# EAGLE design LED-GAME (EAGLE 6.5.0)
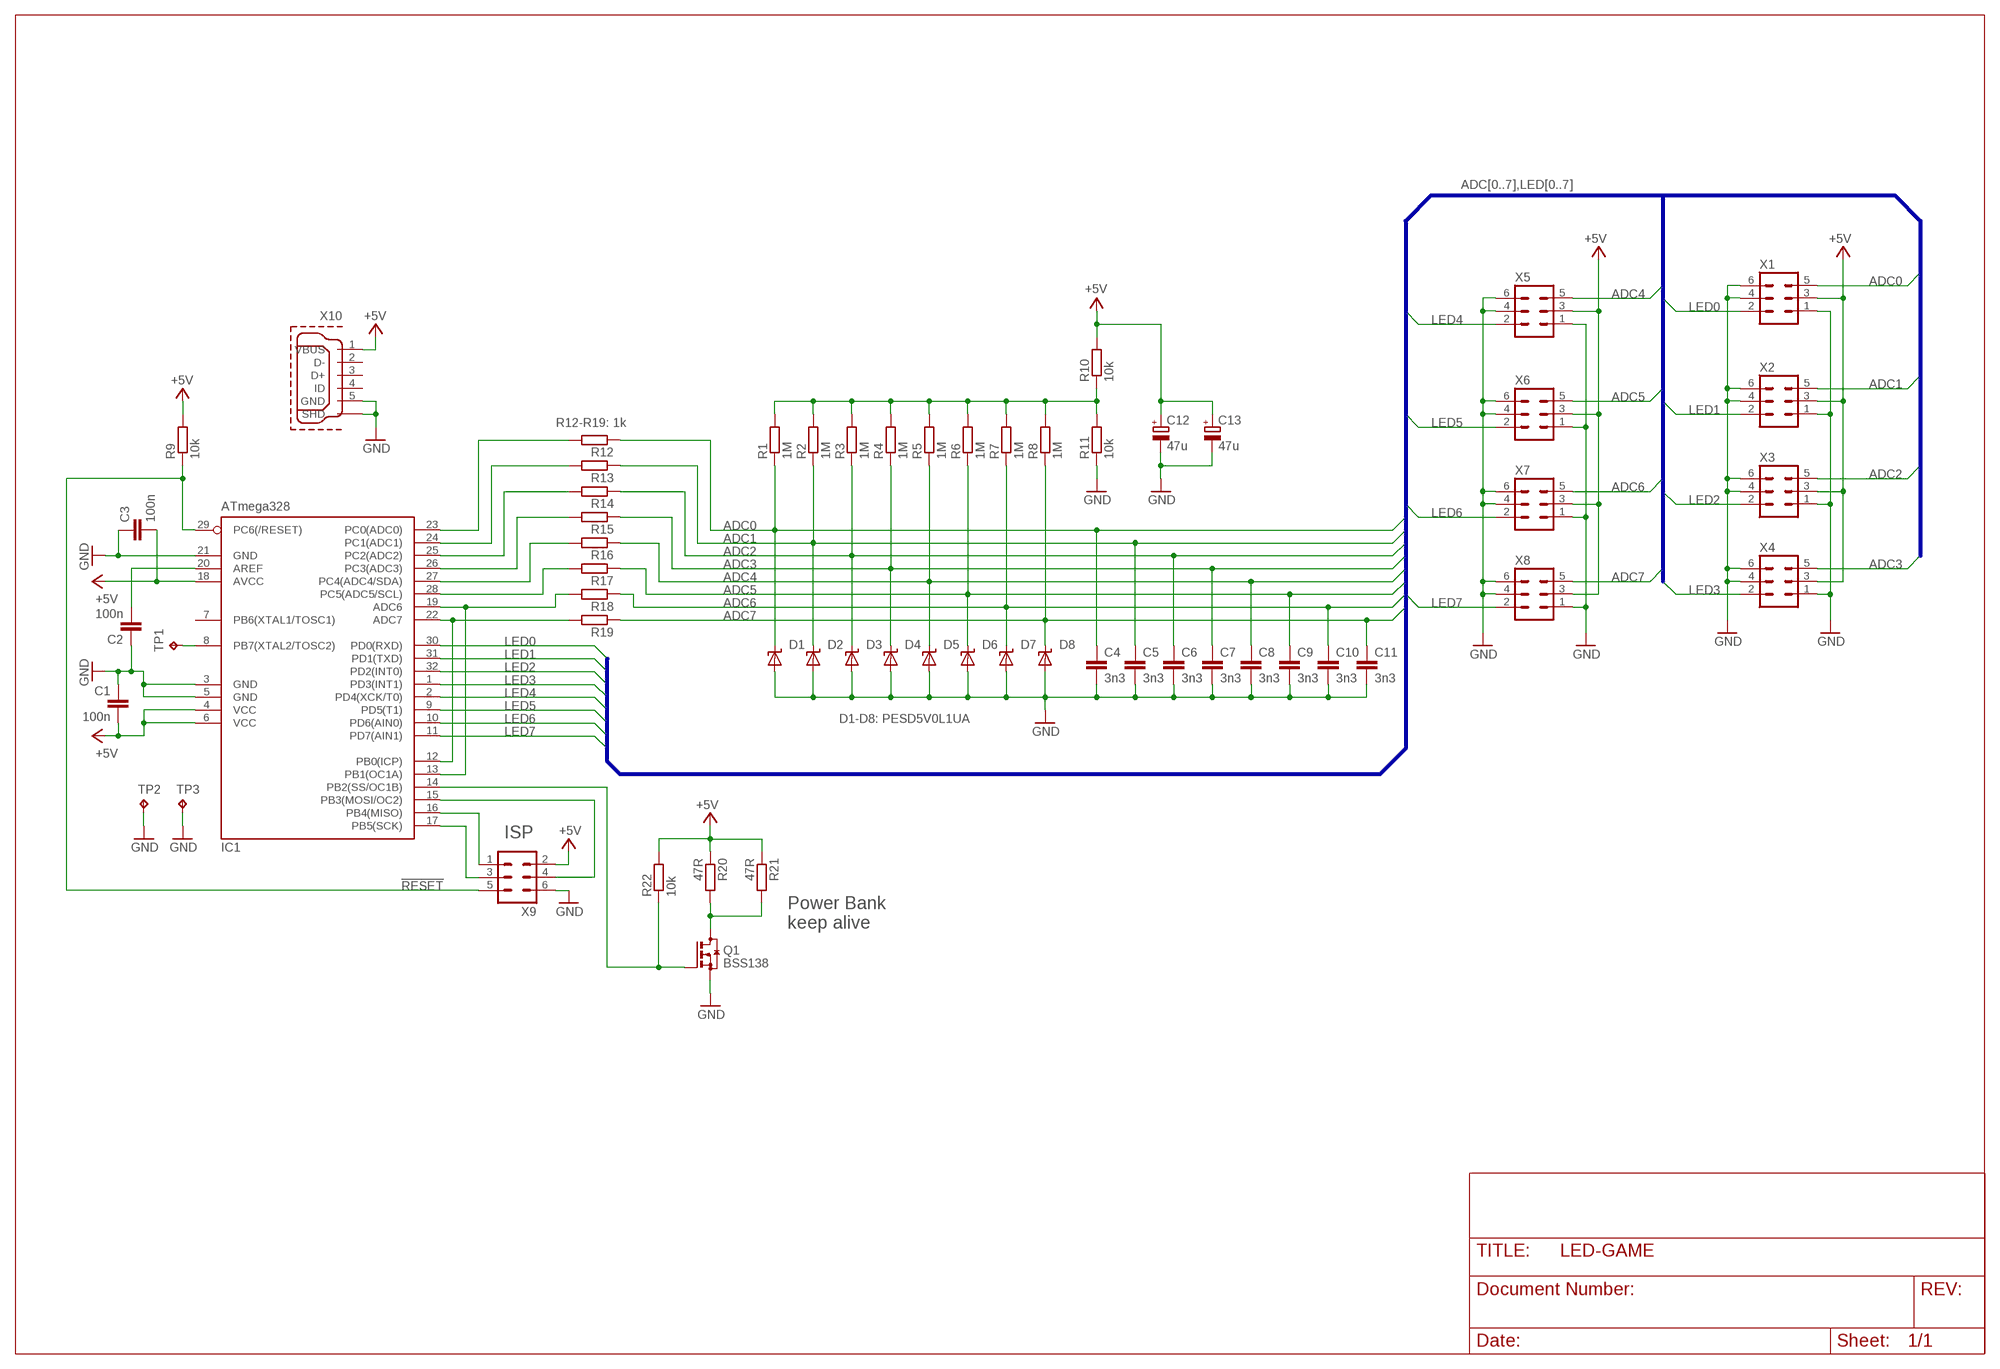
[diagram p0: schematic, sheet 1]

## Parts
C1  100n  C-EUC0603  [C0603]
C2  100n  C-EUC0603  [C0603]
C3  100n  C-EUC0603  [C0603]
C4  3n3  C-EUC0603K  [C0603K]
C5  3n3  C-EUC0603K  [C0603K]
C6  3n3  C-EUC0603K  [C0603K]
C7  3n3  C-EUC0603K  [C0603K]
C8  3n3  C-EUC0603K  [C0603K]
C9  3n3  C-EUC0603K  [C0603K]
C10  3n3  C-EUC0603K  [C0603K]
C11  3n3  C-EUC0603K  [C0603K]
C12  47u  CPOL-EUB/3528-21R  [B/3528-21R]
C13  47u  CPOL-EUB/3528-21R  [B/3528-21R]
D1  PESD5V  SUPPRESSOR_UNI  [SOD323-W]
D2  PESD5V  SUPPRESSOR_UNI  [SOD323-W]
D3  PESD5V  SUPPRESSOR_UNI  [SOD323-W]
D4  PESD5V  SUPPRESSOR_UNI  [SOD323-W]
D5  PESD5V  SUPPRESSOR_UNI  [SOD323-W]
D6  PESD5V  SUPPRESSOR_UNI  [SOD323-W]
D7  PESD5V  SUPPRESSOR_UNI  [SOD323-W]
D8  PESD5V  SUPPRESSOR_UNI  [SOD323-W]
IC1  ATmega328  MEGA8-AI  [TQFP32-08]
Q1  BSS138  BSS123  [SOT23]
R1  1M  R-EU_R0603  [R0603]
R2  1M  R-EU_R0603  [R0603]
R3  1M  R-EU_R0603  [R0603]
R4  1M  R-EU_R0603  [R0603]
R5  1M  R-EU_R0603  [R0603]
R6  1M  R-EU_R0603  [R0603]
R7  1M  R-EU_R0603  [R0603]
R8  1M  R-EU_R0603  [R0603]
R9  10k  R-EU_R0603  [R0603]
R10  10k  R-EU_R0603  [R0603]
R11  10k  R-EU_R0603  [R0603]
R12  1k  R-EU_R0603  [R0603]
R13  1k  R-EU_R0603  [R0603]
R14  1k  R-EU_R0603  [R0603]
R15  1k  R-EU_R0603  [R0603]
R16  1k  R-EU_R0603  [R0603]
R17  1k  R-EU_R0603  [R0603]
R18  1k  R-EU_R0603  [R0603]
R19  1k  R-EU_R0603  [R0603]
R20  47R  R-EU_R1206  [R1206]
R21  47R  R-EU_R1206  [R1206]
R22  10k  R-EU_R0603  [R0603]
TP1  TPP1-08  [P1-08]
TP2  TPP1-08  [P1-08]
TP3  TPP1-08  [P1-08]
X1  ML6  [ML6]
X2  ML6  [ML6]
X3  ML6  [ML6]
X4  ML6  [ML6]
X5  ML6  [ML6]
X6  ML6  [ML6]
X7  ML6  [ML6]
X8  ML6  [ML6]
X9  ML6  [ML6]
X10  MOLEX-1051330001MOD  [MOLEX_1051330001-MOD]

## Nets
!RESET: IC1.29(PC6(/RESET)) R9.1 X9.5
+5V: C1.2 C3.2 C12.+ C13.+ IC1.4(VCC) IC1.6(VCC) IC1.18(AVCC) R9.2 R10.2 R20.1 R21.1 R22.2 X1.3 X2.3 X3.3 X4.3 X5.3 X6.3 X7.3 X8.3 X9.2 X10.1(VBUS)
ADC0: C4.1 D1.C R1.1 R12.1 X1.5
ADC1: C5.1 D2.C R2.1 R13.1 X2.5
ADC2: C6.1 D3.C R3.1 R14.1 X3.5
ADC3: C7.1 D4.C R4.1 R15.1 X4.5
ADC4: C8.1 D5.C R5.1 R16.1 X5.5
ADC5: C9.1 D6.C R6.1 R17.1 X6.5
ADC6: C10.1 D7.C R7.1 R18.1 X7.5
ADC7: C11.1 D8.C R8.1 R19.1 X8.5
GND: C1.1 C2.1 C3.1 C4.2 C5.2 C6.2 C7.2 C8.2 C9.2 C10.2 C11.2 C12.- C13.- D1.A D2.A D3.A D4.A D5.A D6.A D7.A D8.A IC1.3(GND) IC1.5(GND) IC1.21(GND) Q1.2(S) R11.1 TP2.TP TP3.TP X1.1 X1.4 X1.6 X2.1 X2.4 X2.6 X3.1 X3.4 X3.6 X4.1 X4.4 X4.6 X5.1 X5.4 X5.6 X6.1 X6.4 X6.6 X7.1 X7.4 X7.6 X8.1 X8.4 X8.6 X9.6 X10.5(GND) X10.P$1(SHD) X10.P$2(SHD) X10.P$3(SHD) X10.P$5(SHD) X10.P$6(SHD) X10.P$9(SHD)
LED0: IC1.30(PD0(RXD)) X1.2
LED1: IC1.31(PD1(TXD)) X2.2
LED2: IC1.32(PD2(INT0)) X3.2
LED3: IC1.1(PD3(INT1)) X4.2
LED4: IC1.2(PD4(XCK/T0)) X5.2
LED5: IC1.9(PD5(T1)) X6.2
LED6: IC1.10(PD6(AIN0)) X7.2
LED7: IC1.11(PD7(AIN1)) X8.2
N$1: C2.2 IC1.20(AREF)
N$2: IC1.8(PB7(XTAL2/TOSC2)) TP1.TP
N$3: IC1.23(PC0(ADC0)) R12.2
N$4: R1.2 R2.2 R3.2 R4.2 R5.2 R6.2 R7.2 R8.2 R10.1 R11.2
N$5: IC1.24(PC1(ADC1)) R13.2
N$6: IC1.16(PB4(MISO)) X9.1
N$7: IC1.17(PB5(SCK)) X9.3
N$8: IC1.26(PC3(ADC3)) R15.2
N$9: IC1.25(PC2(ADC2)) R14.2
N$10: IC1.27(PC4(ADC4/SDA)) R16.2
N$11: IC1.15(PB3(MOSI/OC2)) X9.4
N$12: IC1.28(PC5(ADC5/SCL)) R17.2
N$13: IC1.14(PB2(SS/OC1B)) Q1.1(G) R22.1
N$14: Q1.3(D) R20.2 R21.2
N$15: IC1.12(PB0(ICP)) IC1.22(ADC7) R19.2
N$16: IC1.13(PB1(OC1A)) IC1.19(ADC6) R18.2
Unconnected: IC1.7(PB6(XTAL1/TOSC1)) X10.2(D-) X10.3(D+) X10.4(ID)

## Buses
ADC[0..7],LED[0..7]

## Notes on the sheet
- R12-R19: 1k
- D1-D8: PESD5V0L1UA
- ISP
- Power Bank
  keep alive

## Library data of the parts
C1-C11 = rcl:C-EU: CAPACITOR, European symbol
C12 C13 = rcl:CPOL-EU: POLARIZED CAPACITOR, European symbol
D1-D8 = Brunner:SUPPRESSOR_UNI
IC1 = atmel:MEGA8: MICROCONTROLLER 8 Kbytes FLASH, 1 kbytes SRAM, 512 bytes EEPROM, USART, 6-channel 10 bit ADC, 2-channel 8 bit ADC Pin compatible with Atmega48, ATMega88, ATMega168 Source: avr.lbr; MPN: ATMEGA8-16AU; OC_FARNELL: 9171371; OC_NEWARK: 73M8863
Q1 = transistor-small-signal:BSS123: N-CHANNEL MOS FET
R1-R22 = rcl:R-EU_: RESISTOR, European symbol
TP1-TP3 = testpad:TP: Test pad
X1-X9 = con-harting-ml:ML6: HARTING; OC_FARNELL: unknown; OC_NEWARK: unknown
X10 = Langloch_cherry:MOLEX-1051330001: USB - Mikro-B Buchsenleiste Steckverbinder 5 Positionen Oberflächenmontage, vertikal

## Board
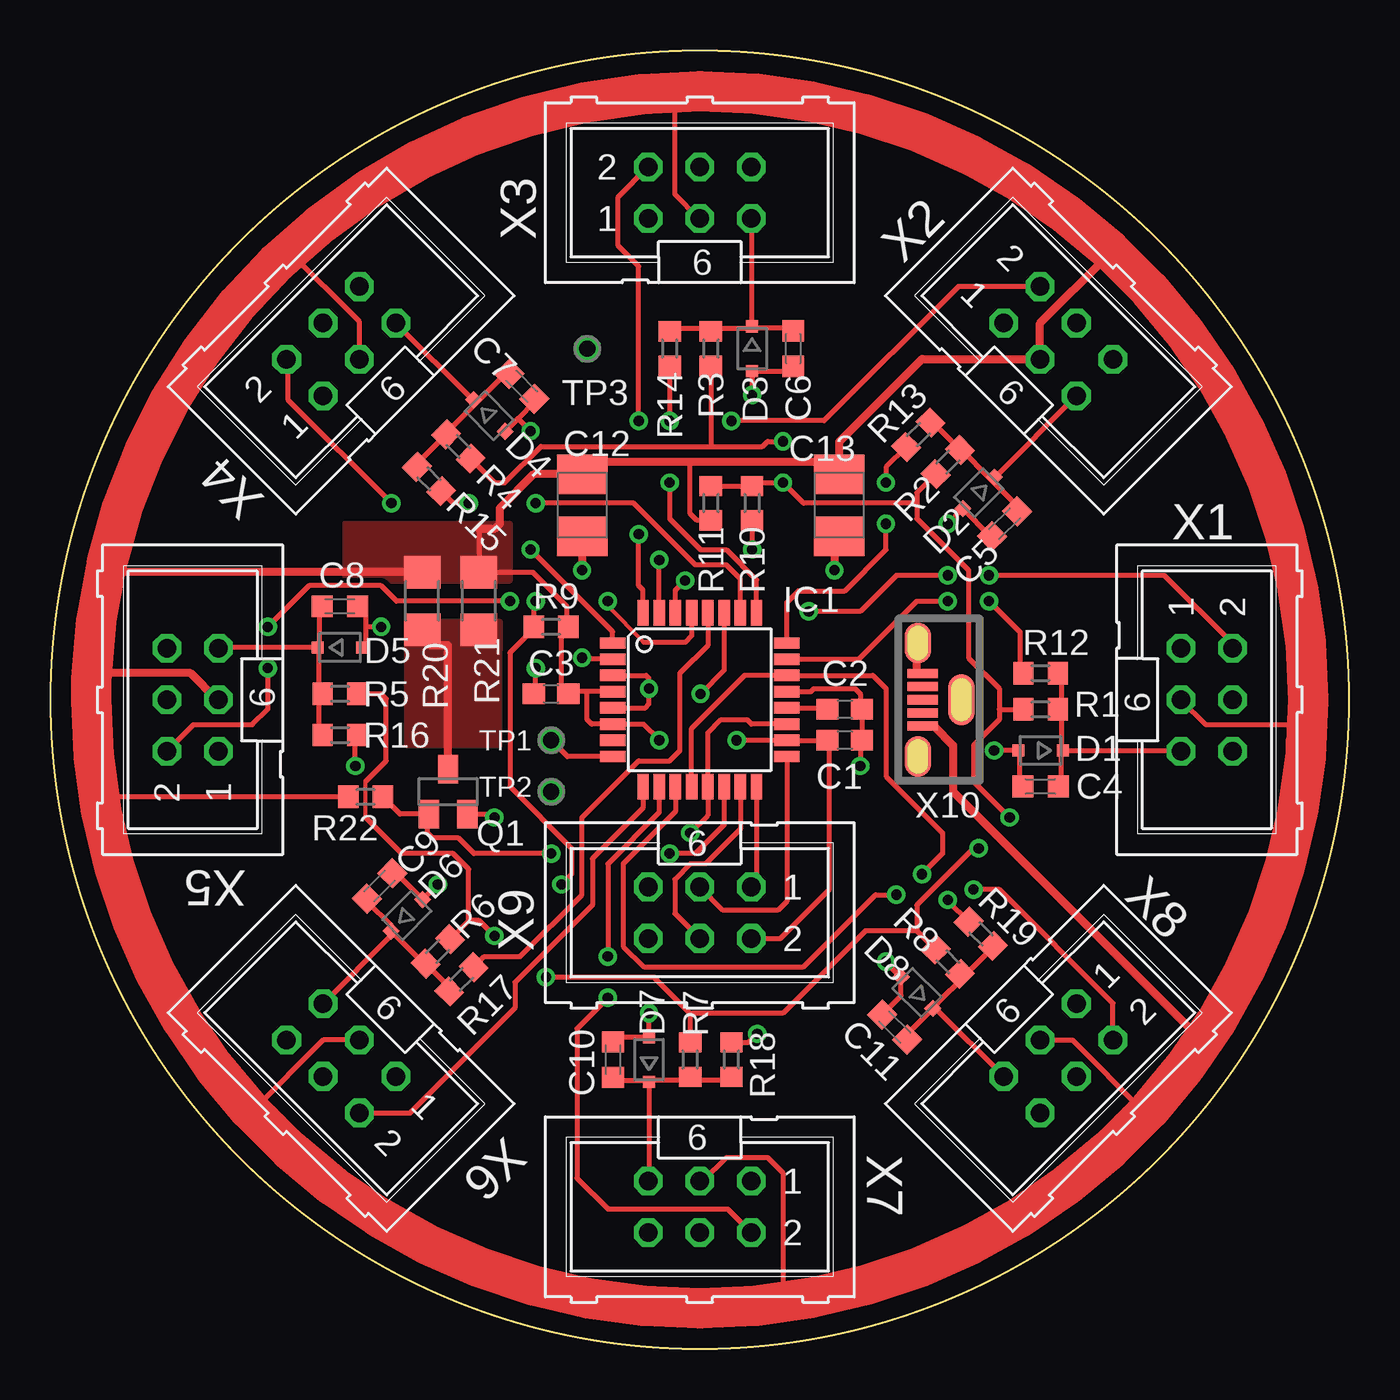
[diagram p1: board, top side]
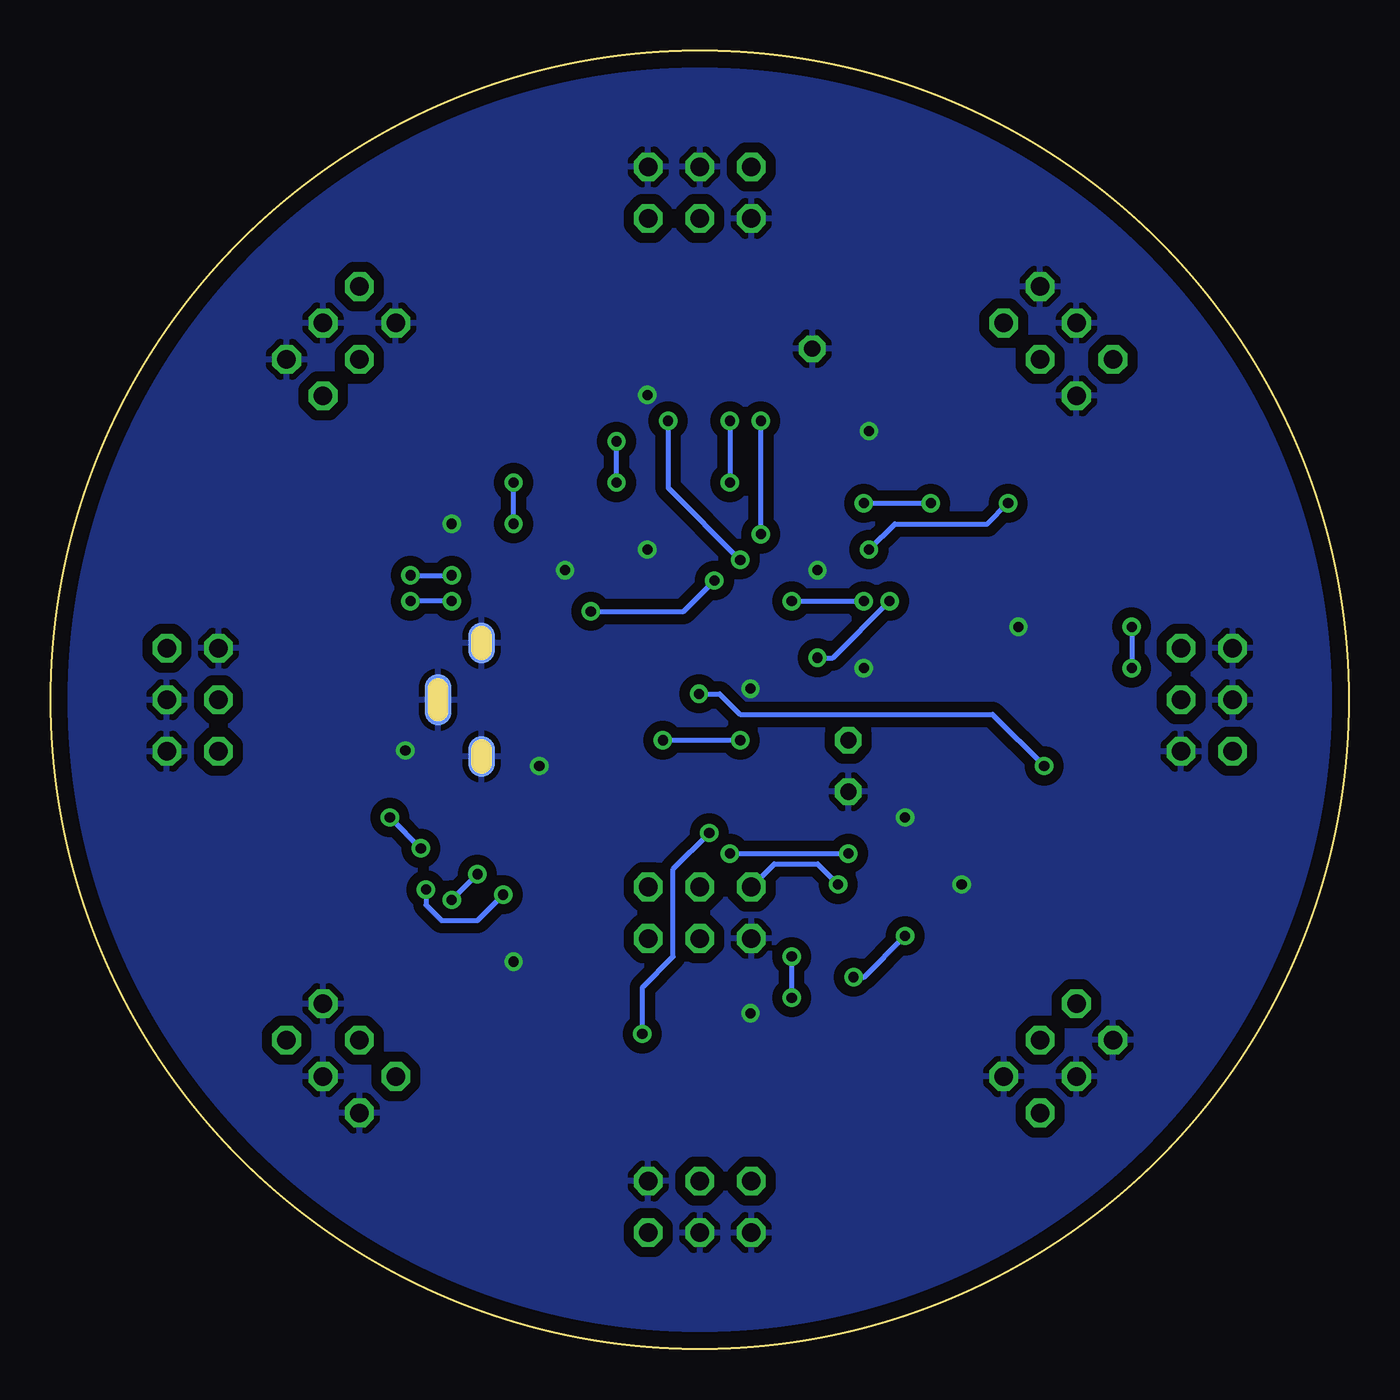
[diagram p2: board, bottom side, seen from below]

Size 64 x 64 mm. Coordinates in mm from the lower left corner, seen from the top.
Outline: circle at 32,32 radius 32
Copper layers (1*16): Top 0.035mm / dielectric 1.5mm / Bottom 0.035mm
Design rules "default *": minimum track width 0.25mm, minimum drill 0.5mm, track to track 0.25mm, track to pad 0.25mm, pad to pad 0.22mm, via to via 0.3mm, smd to smd 8mil, copper to edge 0.8mm, drill to drill 8mil, minimum pad ring 10mil, minimum via ring 8mil, stop-mask expansion 4mil, vias tented up to drill 0mil, thermal gap 0.3mm
bRestrict: 4 lines

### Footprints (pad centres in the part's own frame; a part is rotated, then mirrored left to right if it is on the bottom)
C0603 = smd 1.1 x 1: 1 -0.85,0; 2 0.85,0
C0603K = smd 1.05 x 1.08: 1 -0.875,0; 2 0.875,0
B/3528-21R = smd 1.95 x 2.5: + 1.525,0; - -1.525,0
SOD323-W = smd 0.6 x 0.6: A 1.1,0; C -1.1,0
TQFP32-08 = smd 1.27 x 0.559: 1 -4.293,2.8; 2 -4.293,2; 3 -4.293,1.2; 4 -4.293,0.4; 5 -4.293,-0.4; 6 -4.293,-1.2; 7 -4.293,-2; 8 -4.293,-2.8; 17 4.293,-2.8; 18 4.293,-2; 19 4.293,-1.2; 20 4.293,-0.4; 21 4.293,0.4; 22 4.293,1.2; 23 4.293,2; 24 4.293,2.8 | smd 0.559 x 1.27: 9 -2.8,-4.293; 10 -2,-4.293; 11 -1.2,-4.293; 12 -0.4,-4.293; 13 0.4,-4.293; 14 1.2,-4.293; 15 2,-4.293; 16 2.8,-4.293; 25 2.8,4.293; 26 2,4.293; 27 1.2,4.293; 28 0.4,4.293; 29 -0.4,4.293; 30 -1.2,4.293; 31 -2,4.293; 32 -2.8,4.293
SOT23 = smd 1 x 1.4: 1 -0.95,-1.1; 2 0.95,-1.1; 3 0,1.1
R0603 = smd 1 x 1.1: 1 -0.85,0; 2 0.85,0
R1206 = smd 1.6 x 1.803: 1 -1.422,0; 2 1.422,0
P1-08 = drill 0.8 octagon: TP 0,0
ML6 = drill 0.914 octagon: 1 -2.54,-1.27; 2 -2.54,1.27; 3 0,-1.27; 4 0,1.27; 5 2.54,-1.27; 6 2.54,1.27
MOLEX_1051330001-MOD = smd 1.5 x 0.45: 1 0,1.3; 2 0,0.65; 3 0,0; 4 0,-0.65; 5 0,-1.3 | smd 1.3 x 2 bottom: P$1 0.24,-2.8; P$9 0.24,2.8 | smd 1.3 x 2: P$2 0.24,-2.8; P$3 0.24,2.8 | smd 1.3 x 2.5: P$5 -1.9,0 | smd 1.3 x 2.5 bottom: P$6 -1.9,0

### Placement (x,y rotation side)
C1  39.15,30.01 180 top
C2  39.15,31.53 180 top
C3  24.67,32.29 0 top
C4  48.8,27.72 180 top
C5  47.02,40.67 225 top
C6  36.61,49.31 270 top
C7  23.22,47.46 315 top
C8  14.26,36.61 0 top
C9  16.22,22.82 45 top
C10  27.72,14.26 90 top
C11  41.62,15.86 135 top
C12  26.22,41.59 90 top
C13  38.88,41.59 90 top
D1  48.8,29.5 180 top
D2  45.75,42.2 225 top
D3  34.58,49.31 270 top
D4  21.62,46.01 315 top
D5  14.26,34.58 0 top
D6  17.56,21.37 45 top
D7  29.5,14.26 90 top
D8  42.71,17.56 135 top
IC1  32,32 0 top
Q1  19.59,27.47 0 top
R1  48.8,31.53 180 top
R2  44.23,43.72 225 top
R3  32.55,49.31 270 top
R4  20.1,44.48 315 top
R5  14.26,32.29 0 top
R6  19.08,19.59 45 top
R7  31.53,14.26 90 top
R8  44.23,19.08 135 top
R9  24.67,35.59 0 top
R10  32.55,41.69 270 top
R11  34.58,41.69 90 top
R12  48.8,33.31 180 top
R13  42.78,45.07 225 top
R14  30.51,49.31 270 top
R15  18.65,42.89 315 top
R16  14.26,30.26 0 top
R17  20.25,18.22 45 top
R18  33.56,14.26 90 top
R19  45.86,20.46 135 top
R20  18.32,36.86 270 top
R21  21.12,36.86 270 top
R22  15.53,27.21 180 top
TP1  24.67,30.01 0 top
TP2  24.67,27.47 0 top
TP3  26.45,49.31 0 top
X1  57,32 270 top
X2  49.68,49.68 315 top
X3  32,57 0 top
X4  14.32,49.68 45 top
X5  7,32 90 top
X6  14.32,14.32 135 top
X7  32,7 180 top
X8  49.68,14.32 225 top
X9  32,21.5 180 top
X10  43,32 180 top

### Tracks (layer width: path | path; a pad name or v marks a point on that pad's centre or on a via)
!RESET  (via drill 0.5)
  Top 0.2: 29.24,34.83 27.47,36.61
  Top 0.254: IC1.29 31.6,35.16 31.28,34.83 29.24,34.83 | 27.47,36.61 v27.47,36.86 | v23.91,36.86 23.82,36.78 R9.1 23.82,35.51 22.64,34.32 22.64,27.72 25.69,24.67 25.69,23.4 v25.18,22.89
  Bottom 0.254: v27.47,36.86 v23.91,36.86 | v25.18,22.89 26.2,23.91 28.32,23.91 X9.5
+5V  (via drill 0.5)
  Top 0.254: IC1.4 26.45,32.4 | 26.45,32.4 25.63,32.4 | 25.63,32.4 C3.2 | 26.45,32.4 26.45,31.02 26.67,30.8 IC1.6 29.21,30.8 v30.01,30.01 | C12.+ 26.31,43.21 26.45,43.21 26.96,43.72 | 21.12,40.42 R21.1 23.76,38.29 25.43,36.61 25.43,35.68 R9.2 25.18,35.25 25.18,32.55 25.33,32.4 25.63,32.4 | C13.+ 38.88,43.23 38.39,43.72 | v33.82,30.01 v33.82,30 IC1.18 C1.2 38.39,29.92 38.39,22.64 35.98,20.23 X9.2 | X7.3 32.15,8.27 33.31,9.43 35.34,9.43 36.1,8.67 36.1,2.83 36.36,2.57 32.57,2.57 32,2 | X6.3 13.44,15.22 9.94,11.72 9.94,12.48 6.64,15.78 6.64,16.8 4.35,19.08 4.35,22.13 3.08,23.4 3.08,25.69 2.07,26.7 2.07,27.21 | 2.07,27.21 2.07,31.93 2,32 | X4.3 15.22,50.63 11.72,54.14 12.73,54.14 17.31,58.71 19.08,58.71 20.61,60.23 23.4,60.23 24.67,61.5 28.99,61.5 29.24,61.76 30.77,61.76 | 30.77,61.76 31.76,61.76 32,62 32.24,61.76 37.88,61.76 38.9,60.74 41.44,60.74 42.96,59.22 44.99,59.22 46.52,57.69 48.04,57.69 51.85,53.88 52.1,53.88 | X3.3 31.97,55.73 30.77,56.93 30.77,61.76 | 62.01,32.8 62.01,32.01 62,32 62,31.01 61.76,30.77 | R10.2 31.87,40.84 31.53,41.18 31.53,43.72 | R22.2 2.07,27.21 | X1.3 56.96,30.77 61.76,30.77 | 61.76,30.77 60.99,30.01 60.99,24.93 59.98,23.91 59.98,23.4 | 59.98,22.39 59.47,21.88 59.47,19.59 58.71,18.83 58.71,18.07 57.44,16.8 57.44,16.04 56.68,15.27 55.91,14.51 55.91,13.5 54.14,11.72 53.88,11.72 50.38,15.22 X8.3
  Top 0.406: C12.+ 23.81,43.12 22.13,41.44 22.13,40.67 21.88,40.42 21.12,40.42 | 38.39,43.72 31.53,43.72 26.96,43.72 | R20.1 2.68,38.29 2.57,38.39 2.57,33.57 | 2.57,33.57 2,33 | X5.3 8.2,32 6.89,33.31 2.84,33.31 2.57,33.57 | X2.3 48.78,50.56 52.1,53.88 | 59.98,22.39 59.98,23.4 | 56.68,15.27 44.48,27.47 44.48,29.75 43.54,30.7 X10.1 | C13.+ 38.88,44.72 42.96,48.8 48.8,48.8
  Top 2: 2,32 2,33 arc-88 32,62 arc-90 62,32 arc-90 32,2 arc-90 2,32
  Bottom 0.254: v33.82,30.01 v30.01,30.01
  pour Top (no thermals): 22.64,40.67 14.51,40.67 14.51,37.88 22.64,37.88
ADC0
  Top 0.254: R12.1 49.82,33.31 49.82,31.7 R1.1 49.82,31.53 49.82,29.58 D1.C | D1.C 55.69,29.5 X1.5 | C4.1 49.68,27.83 49.82,27.97 49.82,29.41 D1.C
ADC1
  Top 0.254: R13.1 43.47,45.75 43.47,45.69 R2.1 44.9,44.32 46.26,42.96 | 46.26,42.96 46.52,42.96 D2.C 46.57,42.98 X2.5 | C5.1 47.64,41.58 46.26,42.96
ADC2
  Top 0.254: D3.C 34.58,55.69 X3.5 | R14.1 30.51,50.33 32.38,50.33 R3.1 32.55,50.33 34.49,50.33 D3.C | C6.1 36.61,50.33 34.66,50.33 D3.C
ADC3
  Top 0.254: R15.1 18.05,43.7 18.07,43.72 18.14,43.72 R4.1 19.5,45.15 20.86,46.52 | 20.86,46.52 20.86,46.77 D4.C 20.81,46.79 X4.5 | C7.1 22.42,48.08 20.86,46.52
ADC4
  Top 0.254: 13.5,36.61 C8.1 13.24,36.61 13.24,34.66 D5.C | R16.1 13.41,30.35 13.24,30.51 13.24,32.13 R5.1 13.41,32.38 13.24,32.55 13.24,34.49 D5.C | D5.C 8.31,34.58 X5.5
ADC5
  Top 0.254: R17.1 19.85,17.81 19.66,17.81 R6.1 18.38,18.99 D6.C | C9.1 15.6,22.06 16.8,20.86 16.8,20.61 D6.C | D6.C 16.78,20.37 X6.5
ADC6
  Top 0.254: R18.1 33.56,13.24 31.7,13.24 R7.1 31.44,13.41 31.28,13.24 29.58,13.24 D7.C | C10.1 27.83,13.38 27.97,13.24 29.41,13.24 D7.C | D7.C 29.5,8.31 X7.5
ADC7
  Top 0.254: R19.1 46.46,19.65 46.52,19.59 46.26,19.59 45.25,18.58 44.92,18.58 R8.1 | R8.1 | R8.1 44.99,18.32 43.72,17.05 43.72,17.02 D8.C | C11.1 42.23,15.49 42.2,15.53 42.23,15.53 D8.C | D8.C 43.63,16.78 X8.5
GND  (via drill 0.5)
  Top 0.254: C4.2 47.79,27.72 47.79,29.41 D1.A v46.52,29.5 | v29.5,16.54 D7.A 27.72,15.36 C10.2 | C9.2 17.05,23.44 D6.A v19.08,22.89 | C8.2 15.53,36.61 15.53,35.59 | 15.53,35.59 15.53,34.76 15.36,34.76 D5.A | IC1.3 29.35,33.2 29.5,33.05 v29.5,32.55 29.5,31.78 29.31,31.6 IC1.5 | C3.1 23.82,32.46 23.91,32.55 v23.91,33.56 | C12.- 26.22,39.93 26.2,39.91 | C13.- 38.8,40.07 38.64,39.91 | R11.1 v34.58,39.4 | Q1.2 21.71,26.37 v21.88,26.2 | IC1.21 37.48,32.4 37.63,32.55 39.66,32.55 39.91,32.29 39.91,31.62 C2.1 C1.1 39.91,30.01 v39.91,28.74 | v34.58,47.02 D3.A 36.38,48.21 C6.2 | C5.2 46.34,40.05 D2.A v44.23,40.67 | v16.29,35.59 15.53,35.59 | C11.2 41.93,17.41 D8.A 41.91,18.32 41.18,19.05 v41.18,19.08 | C7.2 23.84,46.67 23.04,45.87 | 23.04,45.87 D4.A | X10.5 42.71,33.3 42.71,33.31 | v23.66,45.25 | v23.66,45.25 23.04,45.87
  Top 0.406: 26.2,39.91 v26.2,38.39 | 38.64,39.91 v38.64,38.39 | 42.71,33.31 42.71,34.75 X10.P$1
  pour Bottom (isolate 0.5): -5.3,69.63 69.63,69.63 69.63,-5.3 -5.3,-5.3
LED0  (via drill 0.5)
  Top 0.254: X1.2 58.27,34.76 54.9,38.13 v46.26,38.13 | v44.23,38.13 41.69,38.13 39.91,36.36 v37.37,36.36 | IC1.30 30.8,37.4 v31.28,37.88
  Bottom 0.254: v46.26,38.13 v44.23,38.13 | v37.37,36.36 32.8,36.36 v31.28,37.88
LED1  (via drill 0.5)
  Top 0.254: X2.2 44.75,52.37 38.13,45.75 v33.56,45.75 | IC1.31 v30,38.89 v30.01,38.9
  Bottom 0.254: v33.56,45.75 33.56,42.45 v30.01,38.9
LED2  (via drill 0.5)
  Top 0.254: IC1.32 29.2,37.42 28.99,37.63 v28.99,40.17 | v28.99,45.75 28.99,53.37 27.97,54.39 27.97,56.78 X3.2
  Bottom 0.254: v28.99,40.17 v28.99,45.75
LED3  (via drill 0.5)
  Top 0.254: IC1.1 27.71,35.35 v23.66,39.4 | v16.8,41.69 11.72,46.77 11.72,48.69 X4.2
  Bottom 0.254: v23.66,39.4 22.39,40.67 17.81,40.67 v16.8,41.69
LED4  (via drill 0.5)
  Top 0.254: IC1.2 26.27,34 v26.2,34.07 | X5.2 7.04,30.77 9.94,30.77 10.7,31.53 v10.7,33.56 | v22.64,36.86 17.05,36.86 16.29,37.63 12.73,37.63 v10.7,35.59
  Bottom 0.254: v26.2,34.07 25.43,34.07 v22.64,36.86 | v10.7,35.59 v10.7,33.56
LED5
  Top 0.254: IC1.9 29.2,26.66 26.7,24.16 26.7,21.88 22.89,18.07 22.89,16.8 17.72,11.63 X6.2
LED6  (via drill 0.5)
  Top 0.254: IC1.10 30,26.44 27.47,23.91 v27.47,19.34 | v27.47,17.31 25.94,15.78 25.94,8.42 27.47,6.89 33.38,6.89 X7.2
  Bottom 0.254: v27.47,19.34 v27.47,17.31
LED7  (via drill 0.5)
  Top 0.254: X8.2 52.37,17.04 46.77,22.64 v45.5,22.64 | IC1.11 30.8,26.48 28.23,23.91 28.23,19.85 29.24,18.83 37.12,18.83 40.67,22.39 v41.69,22.39
  Bottom 0.254: v45.5,22.64 45.5,21.88 44.74,21.12 42.96,21.12 v41.69,22.39
N$1
  Top 0.254: IC1.20 38.23,31.6 C2.2
N$2
  Top 0.254: IC1.8 25.48,29.2 TP1.TP
N$3  (via drill 0.5)
  Top 0.254: IC1.23 39.84,34 42.71,36.86 v44.23,36.86 | v46.26,36.86 47.79,35.34 47.79,33.47 R12.2
  Bottom 0.254: v44.23,36.86 v46.26,36.86
N$4  (via drill 0.5)
  Top 0.2: 15.53,26.2 15.53,27.97
  Top 0.254: R10.1 R11.2 34.67,42.54 34.83,42.71 v36.1,42.71 37.12,41.69 42.71,41.69 | R3.2 32.55,44.48 | 32.55,44.48 35.09,44.48 35.34,44.74 v36.1,44.74 | R2.2 42.71,42.2 42.71,41.69 | 42.71,41.69 42.71,40.93 45.25,38.39 45.25,34.07 46.77,32.55 46.77,31.53 | 42.71,20.61 42.71,21.88 45.5,24.67 v45.75,24.67 | 42.71,20.61 R8.2 | 42.71,20.61 40.17,20.61 36.1,16.54 31.53,16.54 | 31.53,16.54 R7.2 | 31.53,16.54 29.75,18.32 v24.42,18.32 | v21.88,20.35 21.12,21.12 20.61,21.12 | 20.61,21.12 R6.2 | 20.61,21.12 20.61,23.66 19.85,24.42 17.31,24.42 15.53,26.2 | 15.53,27.97 16.54,28.99 16.54,32.04 16.29,32.29 R5.2 | R4.2 | R4.2 21.88,42.71 22.39,42.71 24.16,44.48 32.55,44.48 | 46.77,31.53 R1.2 | 46.77,31.53 46.77,31.02 45.5,29.75 45.5,27.97 v47.28,26.2
  Bottom 0.254: v36.1,42.71 v36.1,44.74 | v24.42,18.32 23.91,18.32 v21.88,20.35 | v47.28,26.2 v45.75,24.67
N$5  (via drill 0.5)
  Top 0.254: IC1.24 36.29,36.8 36.86,37.37 39.15,37.37 41.18,39.4 v41.18,40.67 | R13.2 41.18,43.47 v41.18,42.71
  Bottom 0.254: v41.18,40.67 v41.18,42.71
N$6
  Top 0.254: IC1.16 34.8,23.03 X9.1
N$7
  Top 0.254: IC1.17 36.29,22.07 35.85,21.62 33.15,21.62 X9.3
N$8  (via drill 0.5)
  Top 0.254: IC1.26 34,37.95 33.31,38.64 31.78,38.64 28.74,41.69 v23.91,41.69 | v20.61,41.69 19.85,41.69 R15.2
  Bottom 0.254: v23.91,41.69 v20.61,41.69
N$9  (via drill 0.5)
  Top 0.254: R14.2 v30.51,45.75 | v30.51,42.71 30.51,40.93 32.04,39.4 33.31,39.4 34.8,37.91 IC1.25
  Bottom 0.254: v30.51,45.75 v30.51,42.71
N$10  (via drill 0.5)
  Top 0.254: IC1.27 33.2,33.45 v32.04,32.29 | v15.02,28.74 15.02,30.17 R16.2
  Bottom 0.254: v32.04,32.29 31.02,32.29 30.01,31.28 17.56,31.28 v15.02,28.74
N$11
  Top 0.254: IC1.15 34,25.62 32.29,23.91 31.53,23.91 30.77,23.15 30.77,21.46 X9.4
N$12
  Top 0.254: IC1.28 32.4,34.69 31.02,33.31 31.02,29.5 30.51,28.99 28.99,28.99 26.2,26.2 26.2,22.39 23.15,19.34 21.37,19.34 R17.2
N$13  (via drill 0.5)
  Top 0.254: R22.1 17.22,26.37 Q1.1 18.58,26.3 18.58,25.43 18.83,25.18 20.1,25.18 20.86,24.42 v24.67,24.42 | IC1.14 33.2,25.83 31.78,24.42 v30.51,24.42
  Bottom 0.254: v30.51,24.42 v24.67,24.42
N$14
  Top 0.406: Q1.3 19.59,34.68 18.73,34.68 18.32,35.09 R20.2
  pour Top (no thermals): 17.56,29.75 17.56,35.85 22.13,35.85 22.13,29.75
N$15  (via drill 0.5)
  Top 0.254: IC1.12 31.6,30.58 34.22,33.2 IC1.22 40.53,33.2 41.18,32.55 41.18,28.23 43.98,25.43 43.98,24.42 v42.96,23.4 | v44.23,22.13 44.23,22.09 R19.2
  Bottom 0.254: v42.96,23.4 v44.23,22.13
N$16  (via drill 0.5)
  Top 0.254: R18.2 34.41,15.11 v34.83,15.53 | v31.53,25.43 32.4,26.3 IC1.13 32.4,30.37 33.05,31.02 34.32,31.02 34.55,30.8 IC1.19
  Bottom 0.254: v34.83,15.53 34.83,17.81 33.31,19.34 33.31,23.66 v31.53,25.43

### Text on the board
_tDocu: X3 | X2 | X4 | X1 | X10 | X5 | X8 | X6 | X7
